(* Logix 5000 AddOnInstructionDefinition export AMCI_3601_AOP_Run_Blend; software revision 20.03 *)

ADD_ON_INSTRUCTION AMCI_3601_AOP_Run_Blend   (* revision 0.0, vendor AMCI, ExecuteEnableInFalse *)
// Revision note:
// 3/2020: Version 0 is the initial release
VAR_INPUT
   Axis_Status_Bits : INT; {required}
   Direction_0_Positive_1_Negative : BOOL; {required}
END_VAR
VAR_OUTPUT
   EN : BOOL; {access Read Only, visible}
   ER : BOOL; {access Read Only, visible}
END_VAR
VAR_IN_OUT
   AMCI_3601_output_data : AM:1769_3601:O:0; {required}
END_VAR
VAR
   Upper_Result_X_1000 : DINT;
   command_data_block : INT[10];
        [0]   // Command Bits MSW
        [1]   // Command Bits LSW
        [2]   // Upper Target Position
        [3]   // Lower Target Position
        [4]   // Upper Programmed Speed
        [5]   // Lower Programmed Speed
END_VAR

ROUTINE EnableInFalse   (* ladder *)
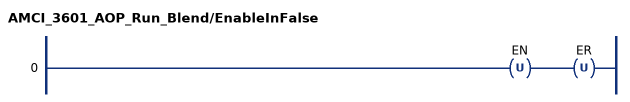
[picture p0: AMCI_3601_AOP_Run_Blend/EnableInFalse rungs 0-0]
   0: OTU(EN)OTU(ER);
END_ROUTINE

ROUTINE Logic   (* ladder *)
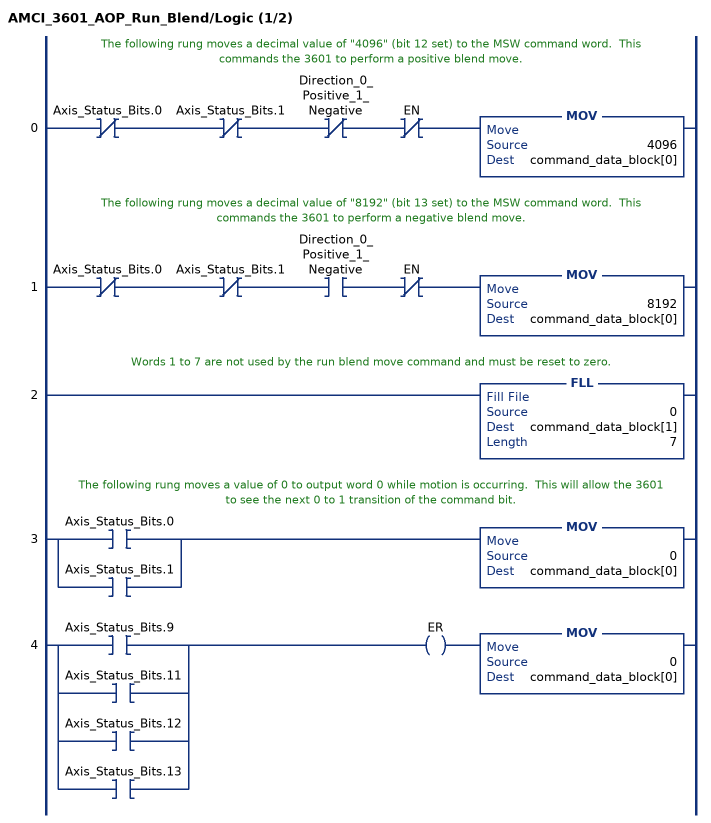
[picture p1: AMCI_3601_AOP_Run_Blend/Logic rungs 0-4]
   // The following rung moves a decimal value of "4096" (bit 12 set) to the MSW command word.  This commands the 3601 to perform a positive blend move.
   0: XIO(Axis_Status_Bits.0)XIO(Axis_Status_Bits.1)XIO(Direction_0_Positive_1_Negative)XIO(EN)MOV(4096,command_data_block[0]);
   // The following rung moves a decimal value of "8192" (bit 13 set) to the MSW command word.  This commands the 3601 to perform a negative blend move.
   1: XIO(Axis_Status_Bits.0)XIO(Axis_Status_Bits.1)XIC(Direction_0_Positive_1_Negative)XIO(EN)MOV(8192,command_data_block[0]);
   // Words 1 to 7 are not used by the run blend move command and must be reset to zero.
   2: FLL(0,command_data_block[1],7);
   // The following rung moves a value of 0 to output word 0 while motion is occurring.  This will allow the 3601 to see the next 0 to 1 transition of the command bit.
   3: [XIC(Axis_Status_Bits.0) ,XIC(Axis_Status_Bits.1) ]MOV(0,command_data_block[0]);
   4: [XIC(Axis_Status_Bits.9) ,XIC(Axis_Status_Bits.11) ,XIC(Axis_Status_Bits.12) ,XIC(Axis_Status_Bits.13) ]OTE(ER)MOV(0,command_data_block[0]);
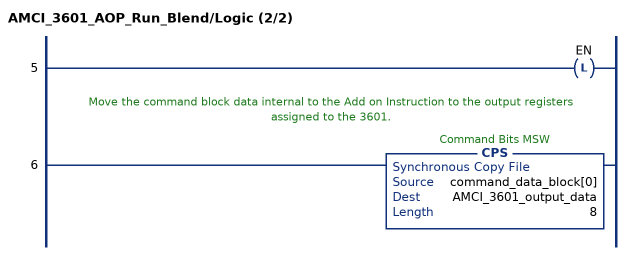
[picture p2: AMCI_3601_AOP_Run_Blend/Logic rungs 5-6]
   5: OTL(EN);
   // Move the command block data internal to the Add on Instruction to the output registers assigned to the 3601.
   6: CPS(command_data_block[0],AMCI_3601_output_data,8);
END_ROUTINE
END_ADD_ON_INSTRUCTION
